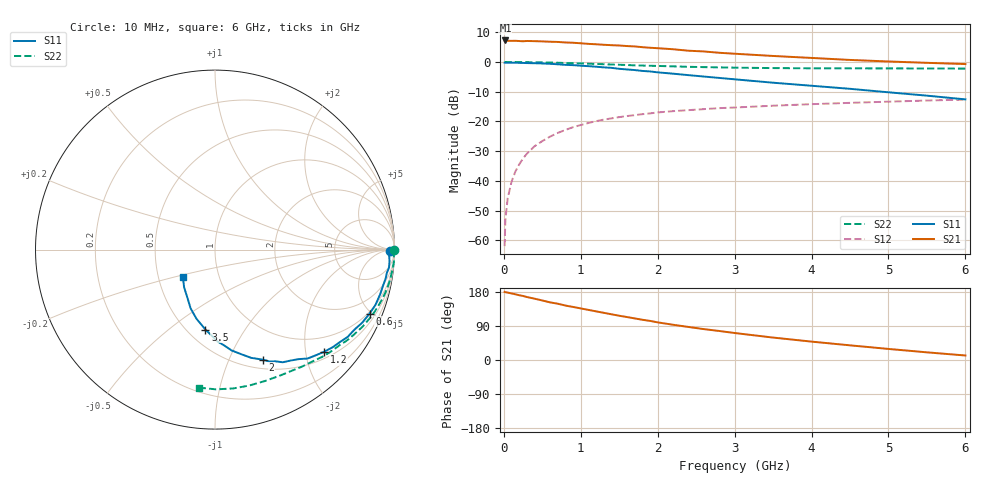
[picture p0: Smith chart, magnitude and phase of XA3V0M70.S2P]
! SIEMENS Discrete & RF Semiconductors
! BFY180
! Si NPN RF Bipolar Junction Transistor in MICRO-X
! VCE = 3 V  IC = 0.7 mA
! Common Emitter S-Parameters:  May  1997
# GHz  S  MA  R  50
!  f  S11  S21  S12  S22
! GHz  MAG  ANG  MAG  ANG  MAG  ANG  MAG  ANG
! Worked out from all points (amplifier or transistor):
!   36 points, 10 MHz to 6 GHz, reference 50 ohm
!   highest |S21| = 7.2 dB at 20 MHz (marker M1)
!   |S21| within 3 dB of that: start of sweep to 2.22 GHz
!   unconditionally stable (mu >= 1): 4.52 GHz to end of sweep
!   at 250 MHz: K = 0.05, MSG = 19.7 dB, |S12| = -32.4 dB
!   at 1.4 GHz: K = 0.44, MSG = 12.3 dB, |S12| = -19.0 dB
!   at 6 GHz: K = 1.04, MAG = 4.7 dB, |S12| = -12.7 dB
!   S11 on the Smith chart (normalised r, x): 10 MHz: 74, -15; 600 MHz: 0.90, -4.87; 1.2 GHz: 0.64, -2.38; 2 GHz: 0.61, -1.34; 3.5 GHz: 0.61, -0.68; 6 GHz: 0.67, -0.22
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0.01  0.9745 -0.3  2.252 179.7  0.0008 87.3  0.9985 -0.2
0.02  0.9711 -0.8  2.302 179.0  0.0022 94.3  0.9999 -0.5
0.05  0.9706 -1.8  2.275 177.9  0.0051 89.9  0.9983 -1.2
0.1  0.9746 -3.9  2.266 175.6  0.0097 89.6  0.9965 -2.5
0.15  0.9747 -5.9  2.273 173.4  0.0144 86.1  0.999 -3.7
0.3  0.959 -11.5  2.256 166.2  0.0288 81.5  0.993 -7.3
0.4  0.9531 -15.2  2.241 161.8  0.0384 79.0  0.9898 -9.7
0.6  0.9321 -22.5  2.191 152.1  0.0555 73.8  0.9782 -14.4
0.9  0.8851 -33.3  2.107 140.0  0.0802 65.1  0.9545 -21.2
1.1  0.8512 -39.8  2.017 132.2  0.0943 60.5  0.9362 -25.4
1.2  0.833 -43.1  1.985 128.3  0.1012 58.0  0.9277 -27.6
1.5  0.7682 -52.6  1.894 116.8  0.1183 51.7  0.8987 -33.3
1.7  0.7323 -59.0  1.827 109.8  0.1276 48.0  0.8774 -36.9
2  0.6693 -66.4  1.705 99.3  0.1418 43.1  0.8583 -41.8
2.2  0.6361 -71.5  1.639 93.0  0.149 39.9  0.8445 -45.1
2.6  0.5691 -80.7  1.505 81.5  0.1611 34.8  0.8195 -50.8
3  0.5115 -88.5  1.377 71.2  0.1715 30.2  0.803 -56.2
3.5  0.4485 -96.8  1.263 59.2  0.1841 25.6  0.79 -62.6
4  0.3984 -105.1  1.17 48.5  0.1953 21.0  0.7834 -69.1
4.5  0.354 -112.6  1.083 38.7  0.2056 16.7  0.7811 -75.8
5.5  0.2717 -129.3  0.968 20.2  0.225 8.4  0.7787 -89.6
6  0.2351 -139.5  0.923 11.9  0.2329 4.0  0.7742 -96.5
